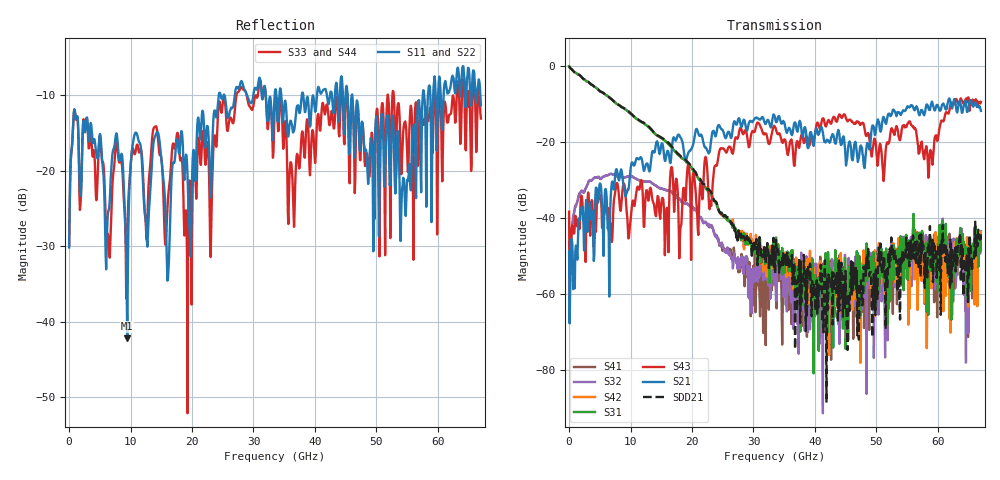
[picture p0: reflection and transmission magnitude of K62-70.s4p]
!Agilent Technologies,N5247A,US50470101,A.10.25.02
!Agilent N5247A: A.10.25.02
!Date: Tuesday, May 12, 2015 13:44:37
!Correction: Sdd11(Full 4 Port(1,2,3,4))
!Sdc11(Full 4 Port(1,2,3,4))
!Sdd12(Full 4 Port(1,2,3,4))
!Sdc12(Full 4 Port(1,2,3,4))
!Scd11(Full 4 Port(1,2,3,4))
!Scc11(Full 4 Port(1,2,3,4))
!Scd12(Full 4 Port(1,2,3,4))
!Scc12(Full 4 Port(1,2,3,4))
!Sdd21(Full 4 Port(1,2,3,4))
!Sdc21(Full 4 Port(1,2,3,4))
!Sdd22(Full 4 Port(1,2,3,4))
!Sdc22(Full 4 Port(1,2,3,4))
!Scd21(Full 4 Port(1,2,3,4))
!Scc21(Full 4 Port(1,2,3,4))
!Scd22(Full 4 Port(1,2,3,4))
!Scc22(Full 4 Port(1,2,3,4))
!Balanced Topology: BBAL
!S4P File: Measurements: <Sdd11,Sdc11,Sdd12,Sdc12>,
!<Scd11,Scc11,Scd12,Scc12>,
!<Sdd21,Sdc21,Sdd22,Sdc22>,
!<Scd21,Scc21,Scd22,Scc22>:
# Hz S  dB  R 50
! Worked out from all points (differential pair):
!   801 points, 10 MHz to 67 GHz, reference 50 ohm
!   strongest paths, dB at 10 MHz, 16.76 GHz, 33.51 GHz, 50.25 GHz, 67 GHz:
!     S21: -48.7, -21.1, -13.6, -14.1, -11.8
!     S43: -38.3, -26.8, -16.0, -25.7, -9.5
!     S31: -0.1, -21.6, -54.0, -59.4, -44.6
!     S42: -0.1, -21.6, -51.7, -51.3, -43.6
!     S32: -46.2, -33.3, -57.2, -53.5, -47.7
!     S41: -49.6, -33.3, -54.8, -47.7, -48.3
!   taken as a pair (ports 1,2 in; 3,4 out), SDD21 dB: -0.1, -21.3, -54.6, -50.9, -43.1
!   lowest |S11| = -42.2 dB at 9.472 GHz (marker M1), VSWR 1.02, Z = 49.3 - j0.255 ohm
!   |S11| at or under -10 dB: start of sweep to 24.35 GHz; 34.52 GHz to 37.87 GHz (3.349 GHz wide, 9.25 % of centre); 46.08 GHz to 57.54 GHz (11.46 GHz wide, 22.1 % of centre)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
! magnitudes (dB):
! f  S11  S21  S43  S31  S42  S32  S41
! 10 MHz  -30.2  -48.7  -38.3  -0.1  -0.1  -46.2  -49.6
! 1.099 GHz  -13.0  -47.2  -39.6  -1.8  -1.8  -36.7  -36.9
! 9.472 GHz  -42.2  -32.9  -39.9  -11.8  -11.8  -29.1  -29.1
! 10.81 GHz  -14.9  -25.1  -34.8  -13.7  -13.7  -29.6  -29.6
! 16.09 GHz  -34.3  -22.4  -43.0  -20.4  -20.4  -32.7  -32.8
! 39.87 GHz  -10.9  -20.2  -19.0  -57.5  -60.7  -57.4  -61.7
! 67 GHz  -11.3  -11.8  -9.5  -44.6  -43.6  -47.7  -48.3
